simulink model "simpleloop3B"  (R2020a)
settings: Solver=ode45  StartTime=0.0  StopTime=10.0  RelTol=1e-3  EnableMultiTasking=on

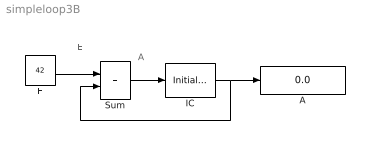
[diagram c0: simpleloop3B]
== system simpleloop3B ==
  note: A
  note: E
  note: .
  A : Display
  E : Constant  Value=42
  IC : InitialCondition  Value=5e17
  Sum : Sum  SaturateOnIntegerOverflow=on
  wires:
  E/1 -> Sum/1
  Sum/1 -> IC/1
  IC/1 -> A/1, Sum/2
